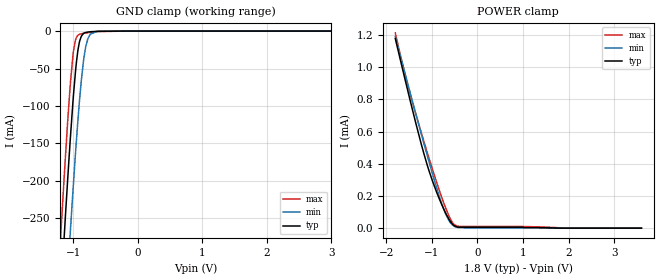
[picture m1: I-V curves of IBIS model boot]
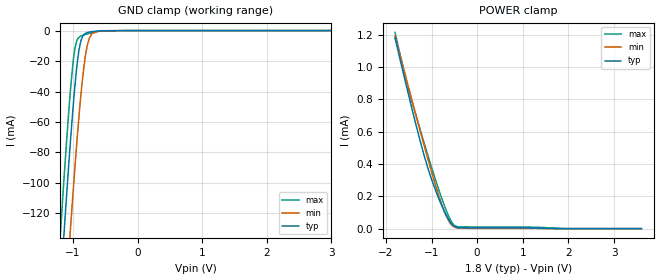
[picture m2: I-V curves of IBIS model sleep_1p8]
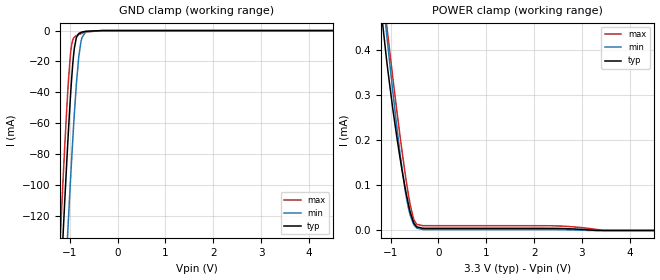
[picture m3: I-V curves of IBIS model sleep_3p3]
|Texas Instruments Incorporated
|Integrated Power Management IC(PMIC) w/4 DC/DCs,8LDOs & RTC in 6x6mm QFN Family
| Marketing part#   Digital Voltage Range   Package-type   #pins
| TPS65910A1RSL   1.8V-5.5V   PVQFN   48
| TPS65910A1RSLR   1.8V-5.5V   PVQFN   48
[IBIS Ver]   4.1
[File name]   tps65910a1.ibs
[File Rev]   1.0
[Date]   9/28/2015
[Source]
| Texas Instruments Incorporated.
| Analog-eLab Design Center, HPA
| 12500 TI Blvd
| Dallas, TX -75243
[Notes]   Revision History:
| Rev 1.0: 9/28/2015
| - Initial version of the model
| - Model generated from simulations in TISPICE
| - Model matched to SPICE simulation
| - C_comp although listed in numerical order of value are
|   obtained from varying PVT conditions. For PVT conditions for
|   each specific value refer the buffer description under
|   respective [Model]. IBIS model user is responsible for using
|   appropriate C_comp to simulate for Signal Integrity.
|* EXCEPTION:   *
|* -For models, boot, sleep_*, pwrhld_*, there are some leakage currents  *
|*  in POWER clamp IV table, because of active pulldown connected to Pad. *
|* -For models, pwron_*  there are some leakage currents in GND clamp IV  *
|*  table, because of active pullup connected to Pad.   *
[Disclaimer]
| This model is designed as an aid for customers of Texas Instruments.
| TI and its licensors and suppliers make no warranties, either expressed
| or implied, with respect to this  model, including the warranties of
| merchantability or fitness for a particular purpose. The model is
| provided solely on an "as is" basis. The entire risk as to its quality
| and performance is with the customer.
[Copyright]
(C) Copyright 2015 Texas Instruments Incorporated.All rights reserved.
|   TPS65910A1RSL
[Component]   TPS65910A1RSL
[Manufacturer]   TI
[Package]   |48 PVQFN - RSL package
|   typ   min   max
R_pkg   0.2   0.16   0.24
L_pkg   1.5nH   1.2nH   1.8nH
C_pkg   0.4pF   0.32pF   0.48pF
[Pin]  signal_name   model_name   R_pin   L_pin   C_pin
1   PWRHOLD   pwrhold   na   na   na
2   VMMC   power   na   na   na
3   VCC3   power   na   na   na
4   VAUX33   power   na   na   na
5   VDIG2   power   na   na   na
6   VCC6   power   na   na   na
7   VDIG1   power   na   na   na
8   SDA   sdascl   na   na   na
9   SCL   sdascl   na   na   na
10   SDASR/EN2   sdascl   na   na   na
11   SCLSR/EN1   sdascl   na   na   na
12   VDDIO   power   na   na   na
13   VCCIO   power   na   na   na
14   SWIO   power   na   na   na
15   GNDIO   gnd   na   na   na
16   VFBIO   nc   na   na   na
17   REFGND   gnd   na   na   na
18   VREF   nc   na   na   na
19   BOOT1   boot   na   na   na
20   OSC32KIN   nc   na   na   na
21   OSC32KOUT   nc   na   na   na
22   VDAC   power   na   na   na
23   VCC5   power   na   na   na
24   VPLL   power   na   na   na
25   TESTV   nc   na   na   na
26   BOOT0   boot   na   na   na
27   VBACKUP   power   na   na   na
28   VCC7   power   na   na   na
29   VRRTC   power   na   na   na
30   VFB3   nc   na   na   na
31   SW3   power   na   na   na
32   VFB1   nc   na   na   na
33   PWRON   pwron   na   na   na
34   GND1   gnd   na   na   na
35   SW1   power   na   na   na
36   VCC1   power   na   na   na
37   SLEEP   sleep   na   na   na
38   CLK32KOUT   clk32kout   na   na   na
39   GPIO/CKSYN   gpio   na   na   na
40   NRESPWRON   nrespwron   na   na   na
41   VCC2   power   na   na   na
42   SW2   power   na   na   na
43   GND2   gnd   na   na   na
44   VFB2   nc   na   na   na
45   INT1   int   na   na   na
46   VAUX1   power   na   na   na
47   VCC4   power   na   na   na
48   VAUX2   power   na   na   na
|   Model Selectors
[Model Selector] sleep
sleep_1p8   1.8V  digital Input
sleep_3p3   3.3V  digital Input
[Model Selector] pwrhold
pwrhld_1p8   1.8V  digital Input
pwrhld_3p3   3.3V  digital Input
pwrhld_5   5.0V  digital Input
[Model Selector] pwron
pwron_1p8   1.8V  digital Input
pwron_3p3   3.3V  digital Input
pwron_5   5.0V  digital Input
[Model Selector] int
int_1p8   1.8V  digital 3-state
int_3p3   3.3V  digital 3-state
[Model Selector] nrespwron
nrespwron_1p8   1.8V  digital 3-state
nrespwron_3p3   3.3V  digital 3-state
[Model Selector] gpio
gpio_1p8   1.8V  digital I/O_open_drain
gpio_3p3   3.3V  digital I/O_open_drain
gpio_5   5.0V  digital I/O_open_drain
[Model Selector] sdascl
sdasclhs_1p8   1.8V  digital I/O_open_drain
sdasclhs_3p3   3.3V  digital I/O_open_drain
sdasclst_1p8   1.8V  digital I/O_open_drain
sdasclst_3p3   3.3V  digital I/O_open_drain
| Models and submodels in the file (21): boot (Input), sleep_1p8 (Input), sleep_3p3 (Input), pwrhld_1p8 (Input), pwrhld_3p3 (Input), pwrhld_5 (Input), pwron_1p8 (Input), pwron_3p3 (Input), pwron_5 (Input), clk32kout (3-state), int_1p8 (3-state), int_3p3 (3-state), nrespwron_1p8 (3-state), nrespwron_3p3 (3-state), gpio_1p8 (I/O_open_drain), gpio_3p3 (I/O_open_drain), gpio_5 (I/O_open_drain), sdasclst_1p8 (I/O_open_drain), sdasclst_3p3 (I/O_open_drain), sdasclhs_1p8 (I/O_open_drain), sdasclhs_3p3 (I/O_open_drain)
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|   boot Model
[Model]   boot
Model_type   Input
Vinl = 0.63
Vinh = 1.17
|   typ   min   max
|   (nom PVT)   (fast PVT)   (slow PVT)
C_comp   7.024e-14   6.987e-14   7.024e-14
[Model spec]
|subparameter
Vinl   0.63   0.5775   0.6825
Vinh   1.17   1.0725   1.2675
| Where nom  PVT is Nominal Process, 1.8V, 27C
|   Fast PVT is Strong Process,  1.95V, -40C
|   Slow PVT is Weak Process,   1.65V, 125C
[Voltage Range]   1.8   1.65   1.95
|Junction Temperature
[Temperature Range]   27   125   -40
[Power Clamp Reference]   1.8   1.65   1.95
[GND Clamp Reference]   0   0   0
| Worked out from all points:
|   GND clamp passes 1 mA (typ) near -0.75 V on its own axis
|   POWER clamp passes 1 mA (typ) near -1.65 V on its own axis
[GND Clamp]
|   Voltage   I(typ)   I(min)   I(max)
-1.8V     -1.31A     -1.432A    -1.238A
-1.204V   -366.1mA   -495.9mA   -286.1mA
-1.151V   -286.8mA   -416.2mA   -207.1mA
-1.121V   -244.8mA   -373.6mA   -165.8mA
-1.043V   -139.3mA   -263.5mA   -67.28mA
-995.4mV  -82.54mA   -199.6mA   -25.17mA
-952.2mV  -41.68mA   -145.8mA   -8.467mA
-908.9mV  -15.89mA   -97.25mA   -4.431mA
-809.4mV  -1.883mA   -21.48mA   -2.56mA
-735.8mV  -890.9uA   -3.998mA   -1.678mA
-626.9mV  -271.5uA   -361.6uA   -641.4uA
3.6V      0A         0A         0A
[POWER Clamp]
|   Voltage   I(typ)   I(min)   I(max)
-1.8V     1.179mA    1.191mA    1.214mA
-1.681V   1.037mA    1.063mA    1.068mA
-1.476V   796.7uA    844.2uA    838uA
-1.231V   523.7uA    586.8uA    595uA
-1.064V   360.1uA    416.1uA    437.8uA
-891mV    222.3uA    248.9uA    283.5uA
-729.1mV  113.9uA    112.4uA    150.9uA
-612mV    50.41uA    42.64uA    69.51uA
-545.4mV  24.73uA    19.51uA    35.1uA
-500.4mV  13.83uA    10.47uA    20.52uA
-418.9mV  6.13uA     3.642uA    11.64uA
3.6V      0A         0A         0A
|   sleep_1p8 Model
[Model]   sleep_1p8
Model_type   Input
Vinl = 0.63
Vinh = 1.17
|   typ   min   max
|   (nom PVT)   (fast PVT)   (slow PVT)
C_comp   7.024e-14   6.994e-14   7.031e-14
[Model spec]
|subparameter
Vinl   0.63   0.5775   0.6825
Vinh   1.17   1.0725   1.2675
| Where nom  PVT is Nominal Process, 1.8V, 27C
|   Fast PVT is Strong Process,  1.95V, -40C
|   Slow PVT is Weak Process,   1.65V, 125C
[Voltage Range]   1.8   1.65   1.95
|Junction Temperature
[Temperature Range]   27   125   -40
[Power Clamp Reference]   1.8   1.65   1.95
[GND Clamp Reference]   0   0   0
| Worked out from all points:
|   GND clamp passes 1 mA (typ) near -0.75 V on its own axis
|   POWER clamp passes 1 mA (typ) near -1.65 V on its own axis
[GND Clamp]
|   Voltage   I(typ)   I(min)   I(max)
-1.8V     -585.1mA   -640.3mA   -553.3mA
-1.193V   -167.5mA   -226.9mA   -131.4mA
-1.139V   -132.4mA   -191.8mA   -96.42mA
-1.056V   -81.54mA   -139.7mA   -47.19mA
-1.035V   -69.53mA   -127.1mA   -36.34mA
-979.2mV  -40.04mA   -94.33mA   -13.84mA
-905.4mV  -12.02mA   -54.89mA   -4.293mA
-852.9mV  -3.858mA   -31.39mA   -3.159mA
-813.6mV  -1.985mA   -17.81mA   -2.614mA
-749mV    -1.004mA   -5.06mA    -1.827mA
-597.1mV  -176.5uA   -203.4uA   -438.8uA
3.6V      0A         0A         0A
[POWER Clamp]
|   Voltage   I(typ)   I(min)   I(max)
-1.8V     1.179mA    1.191mA    1.214mA
-1.681V   1.037mA    1.063mA    1.068mA
-1.476V   796.7uA    844.2uA    838uA
-1.231V   523.7uA    586.8uA    595uA
-1.064V   360.1uA    416.1uA    437.8uA
-891mV    222.3uA    248.9uA    283.5uA
-729.1mV  113.9uA    112.4uA    150.9uA
-612mV    50.41uA    42.64uA    69.51uA
-545.4mV  24.73uA    19.51uA    35.1uA
-500.4mV  13.83uA    10.47uA    20.52uA
-418.9mV  6.13uA     3.642uA    11.64uA
3.6V      0A         0A         0A
|   sleep_3p3 Model
[Model]   sleep_3p3
Model_type   Input
Vinl = 1.155
Vinh = 2.145
|   typ   min   max
|   (nom PVT)   (fast PVT)   (slow PVT)
C_comp   6.081e-14   6.075e-14   6.159e-14
[Model spec]
|subparameter
Vinl   1.155   1.1025   1.2075
Vinh   2.145   2.0475   2.2425
| Where nom  PVT is Nominal Process, 3.3V, 27C
|   Fast PVT is Strong Process,  3.45V, -40C
|   Slow PVT is Weak Process,   3.15V, 125C
[Voltage Range]   3.3   3.15   3.45
|Junction Temperature
[Temperature Range]   27   125   -40
[Power Clamp Reference]   3.3   3.15   3.45
[GND Clamp Reference]   0   0   0
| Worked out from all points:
|   GND clamp passes 1 mA (typ) near -0.75 V on its own axis
|   POWER clamp passes 1 mA (typ) near -1.65 V on its own axis
[GND Clamp]
|   Voltage   I(typ)   I(min)   I(max)
-3.3V     -1.66A     -1.706A    -1.636A
-1.258V   -209.8mA   -269mA     -174mA
-1.147V   -137.7mA   -197mA     -101.6mA
-1.129V   -125.9mA   -185.2mA   -89.95mA
-1.03V    -66.49mA   -123.8mA   -33.7mA
-976.8mV  -38.89mA   -92.97mA   -13.18mA
-900.9mV  -10.93mA   -52.69mA   -4.145mA
-811.5mV  -1.93mA    -17.21mA   -2.587mA
-764.2mV  -1.156mA   -7.034mA   -2.005mA
-663.4mV  -429.8uA   -759.9uA   -944.3uA
-330mV    -3.624uA   -2.417uA   -6.37uA
6.6V      0A         0A         0A
[POWER Clamp]
|   Voltage   I(typ)   I(min)   I(max)
-3.3V     3.033mA    2.855mA    3.247mA
-1.185V   475.6uA    538.9uA    550.8uA
-1.085V   379.4uA    437.5uA    457.6uA
-1.069V   365uA      421.5uA    442.9uA
-871.2mV  208.1uA    230.7uA    266.6uA
-701.3mV  97.31uA    92.78uA    130uA
-590.7mV  41.15uA    33.91uA    57.26uA
-522.8mV  18.57uA    14.37uA    26.81uA
-453.7mV  8.05uA     5.487uA    13.58uA
2.437V    4.579uA    1.886uA    10.22uA
3.448V    0A         0A         30.58nA
6.6V      0A         0A         0A
